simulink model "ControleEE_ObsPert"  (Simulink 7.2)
settings: Solver=ode45  StartTime=0.0  StopTime=50  RelTol=1e-6
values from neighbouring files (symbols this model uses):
  K = acker(A,B,[p p])    [para2nl.m]    (also in para2nl_PI.m = acker(Aa,Ba,[p,p,p]); PrPara2nl_PI.m = acker(Aa,Ba,[p,p,p]); TestesEE.m = acker(A,B,[p,-.6-1.02i,-.6+1.02i]); TestesEEobsPert.m = acker(A,B,[p,-.6-1.0198i,-.6+1.0198i]))
  L = L'    [para2nl.m]    (also in para2nl_PI.m; PrPara2nl_PI.m; TestesEE.m; TestesEEcanalI.m)
  Lc = L(4)    [TestesEEobsPert.m]
  Ls1 = L(5)    [TestesEEobsPert.m]
  Ls2 = L(6)    [TestesEEobsPert.m]
  Nb = gf.den{1}(1,3)/gf.num{1}(1,3)    [para2nl.m]    (also in PrPara2nl_PI.m; TestesEE.m = gf.den{1}(1,4)/gf.num{1}(1,4); TestesEEcanalI.m = -Ki/(100*p); TestesEEobsPert.m = gf.den{1}(1,4)/gf.num{1}(1,4))
  w0 = .5    (= 0.5)    [TestesEEobsPert.m]
libraries: simulink x1

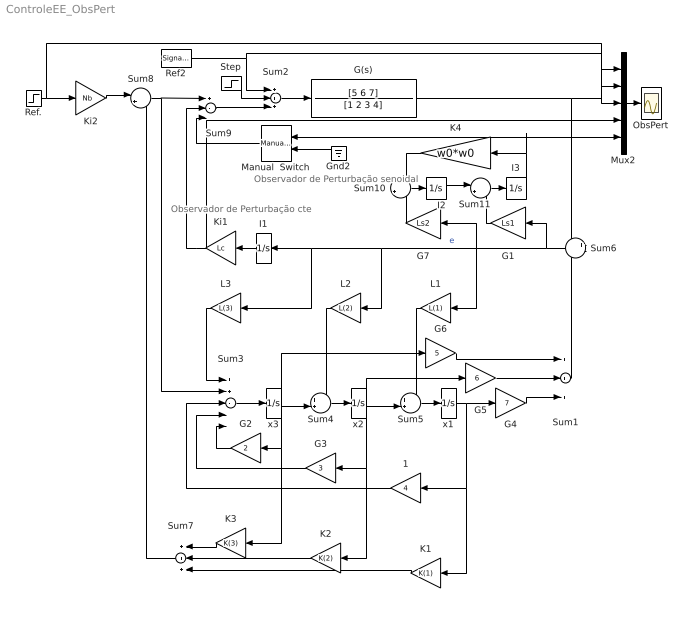
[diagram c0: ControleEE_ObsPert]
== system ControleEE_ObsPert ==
  note: Observador de Perturbação cte
  note: Observador de Perturbação senoidal
  1 : Gain  Orientation=left  Gain=4  ParameterDataType=sfix(16)  ParameterScaling=2^0  OutDataType=sfix(16)  OutScaling=2^0
  G(s) : TransferFcn  Numerator=[5 6 7]  Denominator=[1 2 3 4]
  G1 : Gain  Orientation=left  Gain=Ls1  ParameterDataType=sfix(16)  ParameterScaling=2^0  OutDataType=sfix(16)  OutScaling=2^0
  G2 : Gain  Orientation=left  Gain=2  ParameterDataType=sfix(16)  ParameterScaling=2^0  OutDataType=sfix(16)  OutScaling=2^0
  G3 : Gain  Orientation=left  Gain=3  ParameterDataType=sfix(16)  ParameterScaling=2^0  OutDataType=sfix(16)  OutScaling=2^0
  G4 : Gain  Gain=7  ParameterDataType=sfix(16)  ParameterScaling=2^0  OutDataType=sfix(16)  OutScaling=2^0
  G5 : Gain  Gain=6  ParameterDataType=sfix(16)  ParameterScaling=2^0  OutDataType=sfix(16)  OutScaling=2^0
  G6 : Gain  Gain=5  ParameterDataType=sfix(16)  ParameterScaling=2^0  OutDataType=sfix(16)  OutScaling=2^0
  G7 : Gain  Orientation=left  Gain=Ls2  ParameterDataType=sfix(16)  ParameterScaling=2^0  OutDataType=sfix(16)  OutScaling=2^0
  Gnd2 : Ground  Orientation=left
  I1 : Integrator  Orientation=left
  I2 : Integrator
  I3 : Integrator
  K1 : Gain  Orientation=left  Gain=K(1)  ParameterDataType=sfix(16)  ParameterScaling=2^0  OutDataType=sfix(16)  OutScaling=2^0
  K2 : Gain  Orientation=left  Gain=K(2)  ParameterDataType=sfix(16)  ParameterScaling=2^0  OutDataType=sfix(16)  OutScaling=2^0
  K3 : Gain  Orientation=left  Gain=K(3)  ParameterDataType=sfix(16)  ParameterScaling=2^0  OutDataType=sfix(16)  OutScaling=2^0
  K4 : Gain  Orientation=left  Gain=w0*w0  ParameterDataType=sfix(16)  ParameterScaling=2^0  OutDataType=sfix(16)  OutScaling=2^0
  Ki1 : Gain  Orientation=left  Gain=Lc  ParameterDataType=sfix(16)  ParameterScaling=2^0  OutDataType=sfix(16)  OutScaling=2^0
  Ki2 : Gain  Gain=Nb  ParameterDataType=sfix(16)  ParameterScaling=2^0  OutDataType=sfix(16)  OutScaling=2^0
  L1 : Gain  Orientation=left  Gain=L(1)  ParameterDataType=sfix(16)  ParameterScaling=2^0  OutDataType=sfix(16)  OutScaling=2^0
  L2 : Gain  Orientation=left  Gain=L(2)  ParameterDataType=sfix(16)  ParameterScaling=2^0  OutDataType=sfix(16)  OutScaling=2^0
  L3 : Gain  Orientation=left  Gain=L(3)  ParameterDataType=sfix(16)  ParameterScaling=2^0  OutDataType=sfix(16)  OutScaling=2^0
  Manual  Switch : simulink/Signal Routing/Manual Switch  Orientation=left  SystemSampleTime=-1  sw=1  action=0  varsize=off
  Mux2 : Mux  Inputs=5
  ObsPert : Scope
  Ref. : Step  Time=0  SampleTime=0
  Ref2 : SignalGenerator  Amplitude=.2  Frequency=0.8*w0  Units=rad/sec
  Step : Step  Time=10  After=1.2  SampleTime=0
  Sum1 : Sum  Inputs=+++  OutDataType=sfix(16)  OutScaling=2^0
  Sum10 : Sum  Inputs=-+  OutDataType=sfix(16)  OutScaling=2^0
  Sum11 : Sum  Inputs=|++  OutDataType=sfix(16)  OutScaling=2^0
  Sum2 : Sum  Inputs=+++  OutDataType=sfix(16)  OutScaling=2^0
  Sum3 : Sum  Inputs=++---  OutDataType=sfix(16)  OutScaling=2^0
  Sum4 : Sum  Inputs=++|  OutDataType=sfix(16)  OutScaling=2^0
  Sum5 : Sum  Inputs=++|  OutDataType=sfix(16)  OutScaling=2^0
  Sum6 : Sum  Orientation=left  Inputs=+-  OutDataType=sfix(16)  OutScaling=2^0
  Sum7 : Sum  Orientation=left  Inputs=+++  OutDataType=sfix(16)  OutScaling=2^0
  Sum8 : Sum  Inputs=|+-  OutDataType=sfix(16)  OutScaling=2^0
  Sum9 : Sum  Inputs=+--  OutDataType=sfix(16)  OutScaling=2^0
  x1 : Integrator
  x2 : Integrator
  x3 : Integrator
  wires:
  Ref./1 -> Mux2/1, Ki2/1
  Mux2/1 -> ObsPert/1
  x3/1 -> G6/1, Sum4/2, G2/1, K3/1
  x2/1 -> G5/1, Sum5/2, G3/1, K2/1
  Sum3/1 -> x3/1
  G2/1 -> Sum3/5
  G3/1 -> Sum3/4
  x1/1 -> G4/1, 1/1, K1/1
  1/1 -> Sum3/3
  G4/1 -> Sum1/3
  G5/1 -> Sum1/2
  G6/1 -> Sum1/1
  G(s)/1 -> Sum6/1, Mux2/2
  Sum1/1 -> Sum6/2
  Sum2/1 -> G(s)/1
  Sum4/1 -> x2/1
  Sum5/1 -> x1/1
  Sum6/1 -> L1/1, L2/1, L3/1, I1/1, G7/1, G1/1  "e"
  L3/1 -> Sum3/1
  L2/1 -> Sum4/1
  L1/1 -> Sum5/1
  K3/1 -> Sum7/1
  K2/1 -> Sum7/2
  K1/1 -> Sum7/3
  Sum8/1 -> Sum3/2, Sum9/1
  I1/1 -> Ki1/1
  Ki2/1 -> Sum8/1
  Sum7/1 -> Sum8/2
  I3/1 -> K4/1, Manual  Switch/1, Mux2/5
  Sum10/1 -> I2/1
  Sum11/1 -> I3/1
  K4/1 -> Sum10/1
  I2/1 -> Sum11/1
  G1/1 -> Sum11/2
  G7/1 -> Sum10/2
  Gnd2/1 -> Manual  Switch/2
  Sum9/1 -> Sum2/3
  Step/1 -> Sum2/2
  Ki1/1 -> Sum9/2, Mux2/4
  Ref2/1 -> Mux2/3, Sum2/1
  Manual  Switch/1 -> Sum9/3
